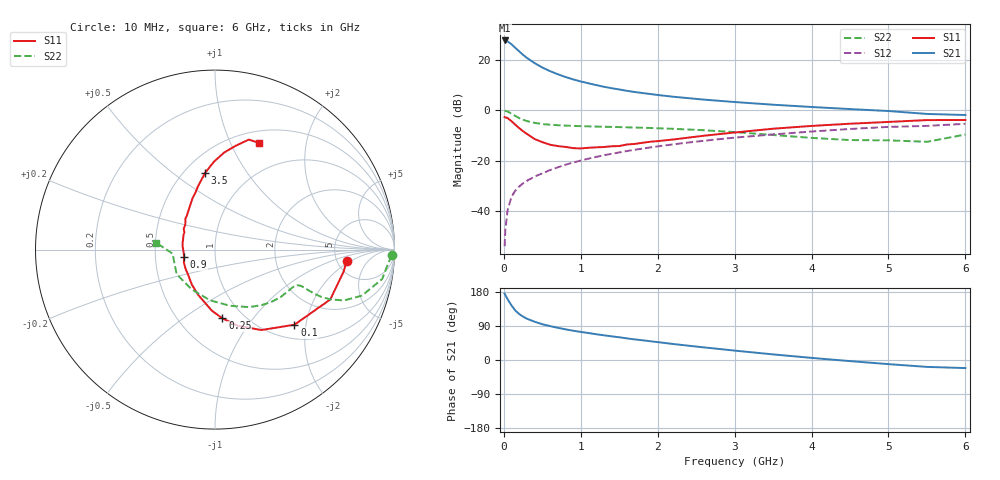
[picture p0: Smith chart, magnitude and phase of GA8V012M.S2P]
! Infineon Technologies  Discrete & RF Semiconductors
! BF775
! Si NPN RF Bipolar Junction Transistor in SOT23
! VCE = 8 V  IC = 12 mA
! Common Emitter S-Parameters:  May  1996
# GHz  S  MA  R  50
!  f  S11  S21  S12  S22
! GHz  MAG  ANG  MAG  ANG  MAG  ANG  MAG  ANG
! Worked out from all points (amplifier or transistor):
!   36 points, 10 MHz to 6 GHz, reference 50 ohm
!   highest |S21| = 27.8 dB at 10 MHz (marker M1)
!   |S21| within 3 dB of that: start of sweep to 151.1 MHz
!   unconditionally stable (mu >= 1): 572.4 MHz to 2.813 GHz
!   at 250 MHz: K = 0.70, MSG = 25.5 dB, |S12| = -29.0 dB
!   at 1.4 GHz: K = 1.09, MAG = 11.2 dB, |S12| = -17.3 dB
!   at 6 GHz: K = 0.89, MSG = 1.7 dB, |S12| = -5.3 dB
!   S11 on the Smith chart (normalised r, x): 10 MHz: 6.10, -1.67; 100 MHz: 1.29, -1.72; 250 MHz: 0.80, -0.72; 900 MHz: 0.70, -0.06; 3.5 GHz: 0.63, +0.66; 6 GHz: 0.64, +1.29
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0.01  0.7358 -4.9  24.53 175.4  0.002 85.8  0.9853 -1.9
0.02  0.7274 -9.6  24.26 171.2  0.0043 85.9  0.9707 -4.1
0.05  0.6999 -23.4  23.45 160.1  0.0106 78.1  0.9456 -10.0
0.1  0.6091 -43.4  20.56 143.8  0.0192 71.4  0.8577 -17.4
0.15  0.5175 -60.0  17.43 130.5  0.0256 66.7  0.7729 -21.5
0.2  0.444 -73.2  14.88 121.4  0.0307 65.0  0.7019 -23.3
0.25  0.3849 -83.9  12.69 114.4  0.0356 63.7  0.6498 -24.0
0.3  0.341 -92.9  11.04 108.9  0.0398 64.6  0.6135 -24.0
0.4  0.2692 -110.4  8.706 101.0  0.0483 65.1  0.5647 -23.5
0.5  0.234 -123.4  7.107 94.4  0.056 66.3  0.5353 -23.0
0.6  0.2078 -135.2  6.033 89.5  0.0651 66.8  0.5189 -22.9
0.7  0.1952 -147.5  5.242 85.0  0.0736 67.0  0.5075 -23.2
0.9  0.1778 -166.0  4.135 77.3  0.0919 67.1  0.491 -24.1
1.1  0.1805 175.9  3.452 71.2  0.1098 66.7  0.4812 -26.0
1.3  0.1868 162.1  2.946 65.2  0.1284 65.6  0.4726 -28.2
1.6  0.21 146.2  2.447 57.0  0.1556 63.6  0.46 -32.3
2.2  0.2637 124.0  1.867 42.3  0.2111 58.7  0.4303 -42.2
2.8  0.3377 108.6  1.549 29.1  0.2678 52.7  0.3859 -54.8
3.5  0.4322 97.2  1.296 14.8  0.3331 44.8  0.324 -75.0
4.5  0.5432 84.6  1.062 -2.9  0.427 32.4  0.257 -120.4
5.5  0.6413 72.9  0.85 -18.2  0.4916 17.4  0.2373 -174.6
6  0.6433 67.4  0.809 -21.3  0.541 13.3  0.3312 173.2
